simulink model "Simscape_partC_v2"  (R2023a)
settings: Solver=VariableStepAuto  StartTime=0.0  StopTime=5  FixedStep=1/(490*4)  RelTol=1e-3
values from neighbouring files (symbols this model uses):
  Ki = 250    [project_constants.m]
  Kp = 250    [project_constants.m]
  theta_des = pi/2    (= 1.57079632679)    [project_constants.m]
libraries: fl_lib x5, nesl_utility x5, ee_lib x4, simulink x2

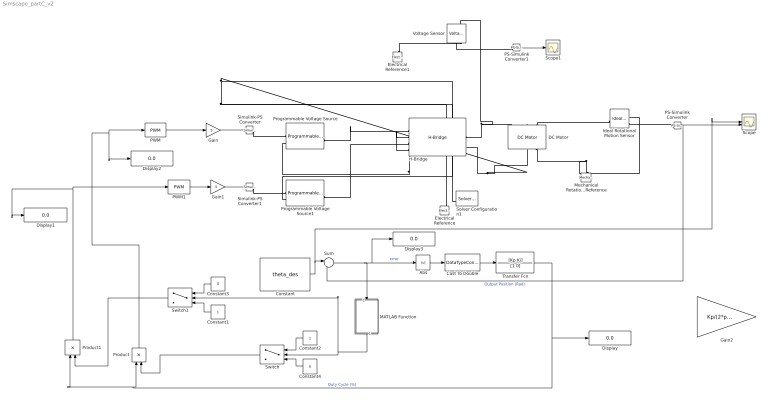
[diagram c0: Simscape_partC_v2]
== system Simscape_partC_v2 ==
  Abs : Abs
  Cast To Double : DataTypeConversion  OutDataTypeStr=double
  Constant : Constant  Value=theta_des
  Constant1 : Constant
  Constant2 : Constant
  Constant3 : Constant  Value=0
  Constant4 : Constant  Value=0
  DC Motor : ee_lib/Electromechanical/Brushed Motors/DC Motor  field_option=ee.enum.field_option.pm  Rf=100 Ohm  Lf=1 H  Laf=0.15 H  If0=0 A  parameterization=ee.enum.dcparam_option.circuit_param  Ra=5 Ohm  La=12e-6 H  emf_or_torque=ee.enum.emf_or_torque.ki  Kv=6/35 V/rpm  Ki=.1032 N*m/A  T_stall=140*9.81/1000 N*m  w_max=35 rpm  w_rated=15000 rpm  P_rated=0.08 W  V_rated=6 V  lam_param=ee.enum.lam_param.damping  i_noload=0 A  V_i_noload=1.5 V  J=9.76e-3 kg*m^2  lam=b N*m*s/rad  speed0=0 rpm  enable_fault_armature=simscape.enum.onoff.off  rev_faulted=1 / 3  G_faulted_armature=1e-5 S  fault_trigger_armature=ee.enum.faults.faultTrigger.temporal  t_fault_armature=1 s  max_permissible_current_armature=inf A  t_fail_on_current_armature=1 s  enable_fault_field=simscape.enum.onoff.off  G_faulted_field=1e-5 S  fault_trigger_field=ee.enum.faults.faultTrigger.temporal  t_fault_field=1 s  max_permissible_current_field=inf A  t_fail_on_current_field=1 s  fault_action=simscape.enum.assert.action.none  alpha=3.93e-3 1/K  Tmeas=25 degC  thermal_mass=100 J/K  initial_temperature=25 degC
  Display{,1..3} (4 alike) : Display
  Electrical Reference : fl_lib/Electrical/Electrical Elements/Electrical Reference
  Electrical Reference1 : fl_lib/Electrical/Electrical Elements/Electrical Reference
  Gain : Gain  Gain=5
  Gain1 : Gain  Gain=5
  Gain2 : Gain  Gain=Kp/(2*pi)
  H-Bridge : ee_lib/Semiconductors & Converters/Converters/H-Bridge  supply_ports=ee.enum.supply_ports.hidesupply  pwm_or_av=ee.enum.pwm_or_av.averaged  regenerative_braking_mode=ee.enum.converters.regenerative_braking_mode.depends_on_rev  discontinuous=ee.enum.current_profile.continuous  freewheeling_mode=ee.enum.converters.freewheeling_mode.one_switch_one_diode  Rload=10 Ohm  Lload=1e-5 H  F=10 kHz  Venable=2.5 V  Vmax=5 V  Vreverse=.1 V  Vbrake=.1 V  Vm=7.5 V  Ron=0.1 Ohm  Don=0.05 Ohm  Goff=1e-6 S  Tmeas=298.15 K  Ron2=0.1 Ohm  Don2=0.05 Ohm  Tmeas2=398.15 K  thermal_mass=100 J/K  initial_temperature=298.15 K
  Ideal Rotational Motion Sensor : fl_lib/Mechanical/Mechanical Sensors/Ideal Rotational Motion Sensor  reference=foundation.enum.MeasurementReference.difference  acceleration_port=false  velocity_port=true  position_port=true  wrap_angle=false  offset=0 rad
  MATLAB Function : MATLAB Function  TreatAsAtomicUnit=on
  Mechanical Rotational Reference : fl_lib/Mechanical/Rotational Elements/Mechanical Rotational Reference
  PS-Simulink Converter : nesl_utility/PS-Simulink Converter  PhysicalDomain=network_engine_domain  SubClassName=ps_output  LeftPortType=input  RightPortType=output  PseudoPeriodic=off  Frequencies=[]  VectorFormat=inherit  Unit=inherit  AffineConversion=off
  PS-Simulink Converter1 : nesl_utility/PS-Simulink Converter  PhysicalDomain=network_engine_domain  SubClassName=ps_output  LeftPortType=input  RightPortType=output  PseudoPeriodic=off  Frequencies=[]  VectorFormat=inherit  Unit=inherit  AffineConversion=off
  PWM : simulink/Discontinuities/PWM  DisableCoverage=on  Period=1/490  InitialDelay=0  DisallowZeroDutyCycle=off  RunAtFixedTimeIntervals=off  SampleTime=1/(490*2)
  PWM1 : simulink/Discontinuities/PWM  DisableCoverage=on  Period=1/490  InitialDelay=0  DisallowZeroDutyCycle=off  RunAtFixedTimeIntervals=off  SampleTime=1/(490*2)
  Product : Product
  Product1 : Product
  Programmable Voltage Source : ee_lib/Sources/Programmable Voltage Source  magnitude_type=ee.enum.timechanging.constant  ac_magnitude=0 V  magn_ramp=1 V/s  magn_step=1 V  magn_modu_magn=1 V  magn_modu_freq=1 Hz  magn_t1=1 s  magn_t2=2 s  frequency_type=ee.enum.timechanging.constant  ac_frequency=60 Hz  freq_ramp=1 Hz/s  freq_step=1 Hz  freq_modu_magn=1 Hz  freq_modu_freq=1 Hz  freq_t1=1 s  freq_t2=2 s  phase_type=ee.enum.timechanging.constant  ac_shift=0 deg  phase_ramp=1 deg/s  phase_step=1 deg  phase_modu_magn=1 deg  phase_modu_freq=1 Hz  phase_t1=1 s  phase_t2=2 s  dc_type=ee.enum.timechanging.external  dc_voltage=0 V  dc_ramp=1 V/s  dc_step=1 V  dc_modu_magn=1 V  dc_modu_freq=1 Hz  dc_t1=1 s  dc_t2=2 s  harmonic_option=0  harmonic_orders=[5, 7, 11, 13]  harmonic_ratios=[.1, .1, .1, .1]  harmonic_shifts=[0, 0, 0, 0] deg  harmonic_t1=-inf s  harmonic_t2=inf s  noise_mode=0  PSD=0 V^2/Hz  repeatability=1  auto_seed=0  user_seed=0  sample_time=1e-3 s  i_specify=off  i_priority=None  i=0 A  i_nominal_specify=off  i_nominal_unit=A  i_nominal_value=1  v_specify=off  v_priority=None  v=0 V  v_nominal_specify=off  v_nominal_unit=V  v_nominal_value=1
  Programmable Voltage Source1 : ee_lib/Sources/Programmable Voltage Source  magnitude_type=ee.enum.timechanging.constant  ac_magnitude=0 V  magn_ramp=1 V/s  magn_step=1 V  magn_modu_magn=1 V  magn_modu_freq=1 Hz  magn_t1=1 s  magn_t2=2 s  frequency_type=ee.enum.timechanging.constant  ac_frequency=60 Hz  freq_ramp=1 Hz/s  freq_step=1 Hz  freq_modu_magn=1 Hz  freq_modu_freq=1 Hz  freq_t1=1 s  freq_t2=2 s  phase_type=ee.enum.timechanging.constant  ac_shift=0 deg  phase_ramp=1 deg/s  phase_step=1 deg  phase_modu_magn=1 deg  phase_modu_freq=1 Hz  phase_t1=1 s  phase_t2=2 s  dc_type=ee.enum.timechanging.external  dc_voltage=0 V  dc_ramp=1 V/s  dc_step=1 V  dc_modu_magn=1 V  dc_modu_freq=1 Hz  dc_t1=1 s  dc_t2=2 s  harmonic_option=0  harmonic_orders=[5, 7, 11, 13]  harmonic_ratios=[.1, .1, .1, .1]  harmonic_shifts=[0, 0, 0, 0] deg  harmonic_t1=-inf s  harmonic_t2=inf s  noise_mode=0  PSD=0 V^2/Hz  repeatability=1  auto_seed=0  user_seed=0  sample_time=1e-3 s  i_specify=off  i_priority=None  i=0 A  i_nominal_specify=off  i_nominal_unit=A  i_nominal_value=1  v_specify=off  v_priority=None  v=0 V  v_nominal_specify=off  v_nominal_unit=V  v_nominal_value=1
  Scope : Scope  NumInputPorts=2
  Scope1 : Scope
  Simulink-PS Converter : nesl_utility/Simulink-PS Converter  PhysicalDomain=network_engine_domain  SubClassName=ps_input  LeftPortType=input  RightPortType=output  PseudoPeriodic=off  Frequencies=[]  NoiseDistribution=none  NoiseParameters=[]  Unit=1  AffineConversion=off  FilteringAndDerivatives=provide  SimscapeFilterOrder=1  InputFilterTimeConstant=0.001  UdotUserProvided=0
  Simulink-PS Converter1 : nesl_utility/Simulink-PS Converter  PhysicalDomain=network_engine_domain  SubClassName=ps_input  LeftPortType=input  RightPortType=output  PseudoPeriodic=off  Frequencies=[]  NoiseDistribution=none  NoiseParameters=[]  Unit=1  AffineConversion=off  FilteringAndDerivatives=provide  SimscapeFilterOrder=1  InputFilterTimeConstant=0.001  UdotUserProvided=0
  Solver Configuration1 : nesl_utility/Solver Configuration  PhysicalDomain=network_engine_domain  SubClassName=solver  LeftPortType=input  RightPortType=generic  Tones=[]  Harmonics=[]  SimulateNoise=off  Profile=off  UseLocalSampling=off  EnableSwitchedLinearOptims=on  FrequencyDomain=off  UseCCode=off  RelTol=0.001  AbsTol=0.001  MinStep=1e-09  ToWorkspace=off  RevertToSquareIcSolve=off  NumHomotopyIterations=100  PhasorMode=off  PhasorModeNumHarmonics=1  ConsistencySolver=NEWTON_XTOL_AFTER_FTOL  IndexReductionMethod=DerivativeReplacement  DoDC=off  ResidualTolerance=1e-09  ConsistencyTolSource=GLOBAL  ConsistencyAbsTol=0.001  ConsistencyRelTol=0.001  ConsistencyTolFactor=0.001  UseLocalSolver=off  LocalSolverChoice=NE_BACKWARD_EULER_ADVANCER  ResolveIndetEquations=on  FunctionEvalNumThread=1  LocalSolverSampleTime=0.001  DoFixedCost=off  MaxNonlinIter=3  MaxModeIter=2  ComputeImpulses=off  ImpulseIterations=2  LinearAlgebra=auto  LinearAlgebraNumThread=0  EquationFormulation=NE_TIME_EF  DelaysMemoryBudget=1024  AutomaticFiltering=on  FilteringTimeConstant=0.001  PartitionStorageMethod=AS_NEEDED  PartitionMemoryBudget=1024  PartitionMethod=ROBUST
  Sum : Sum  Inputs=|+-
  Switch : Switch  Criteria=u2 > Threshold
  Switch1 : Switch  Criteria=u2 > Threshold
  Transfer Fcn : TransferFcn  Numerator=[Kp Ki]  Denominator=[1 0]
  Voltage Sensor : fl_lib/Electrical/Electrical Sensors/Voltage Sensor
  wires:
  Transfer Fcn/1 -> Product1/1, Product/1, Display/1  "Duty Cycle (%)"
  PS-Simulink Converter/1 -> Sum/2, Scope/2  "Output Position (Rad)"
  PWM/1 -> Gain/1
  Gain/1 -> Simulink-PS Converter/1
  Constant/1 -> Scope/1, Sum/1
  Sum/1 -> Display3/1, Abs/1, MATLAB Function/1(u)  "error"
  Abs/1 -> Cast To Double/1
  Gain1/1 -> Simulink-PS Converter1/1
  PWM1/1 -> Gain1/1
  MATLAB Function/1(y) -> Switch1/2, Switch/2
  Constant4/1 -> Switch/3
  Constant2/1 -> Switch/1
  Switch/1 -> Product/2
  Constant1/1 -> Switch1/3
  Constant3/1 -> Switch1/1
  Switch1/1 -> Product1/2
  Product1/1 -> PWM1/1, Display1/1
  Product/1 -> Display2/1, PWM/1
  PS-Simulink Converter1/1 -> Scope1/1
  Cast To Double/1 -> Transfer Fcn/1
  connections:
  H-Bridge/RConn1 -- DC Motor/LConn1 -- Voltage Sensor/LConn1
  DC Motor/RConn2 -- Ideal Rotational Motion Sensor/RConn1 -- Mechanical Rotational Reference/LConn1
  DC Motor/LConn2 -- Ideal Rotational Motion Sensor/LConn1
  Simulink-PS Converter/RConn1 -- Programmable Voltage Source/RConn1
  PS-Simulink Converter/LConn1 -- Ideal Rotational Motion Sensor/RConn3
  H-Bridge/LConn4 -- Programmable Voltage Source1/RConn2 -- Solver Configuration1/RConn1 -- Electrical Reference/LConn1 -- DC Motor/RConn1 -- H-Bridge/RConn2 -- Programmable Voltage Source/RConn2 -- H-Bridge/LConn2
  Programmable Voltage Source/LConn1 -- H-Bridge/LConn1
  Programmable Voltage Source1/LConn1 -- H-Bridge/LConn3
  Simulink-PS Converter1/RConn1 -- Programmable Voltage Source1/RConn1
  Electrical Reference1/LConn1 -- Voltage Sensor/RConn2
  Voltage Sensor/RConn1 -- PS-Simulink Converter1/LConn1

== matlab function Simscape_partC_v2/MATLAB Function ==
function y = fcn(u)

y = u/abs(u);
